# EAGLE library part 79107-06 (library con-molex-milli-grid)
RECEPTACAL
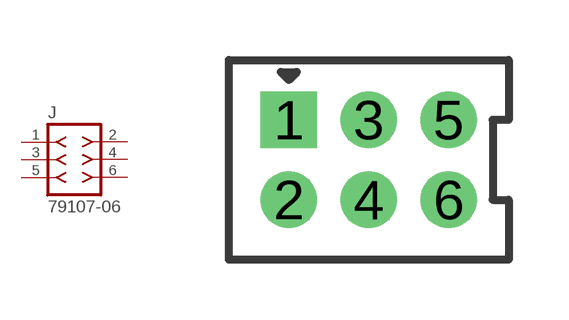
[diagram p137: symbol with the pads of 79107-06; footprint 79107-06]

Designator prefix J

## 79107-06  [79107-06]
1  1  pas
2  2  pas
3  3  pas
4  4  pas
5  5  pas
6  6  pas

## Footprint 79107-06 (pad centres in mm)
RECEPTACAL Dual Row, Vertical, Through-Hole
drill 0.914 square: 1 -2,1
drill 0.914: 2 -2,-1; 3 0,1; 4 0,-1; 5 2,1; 6 2,-1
